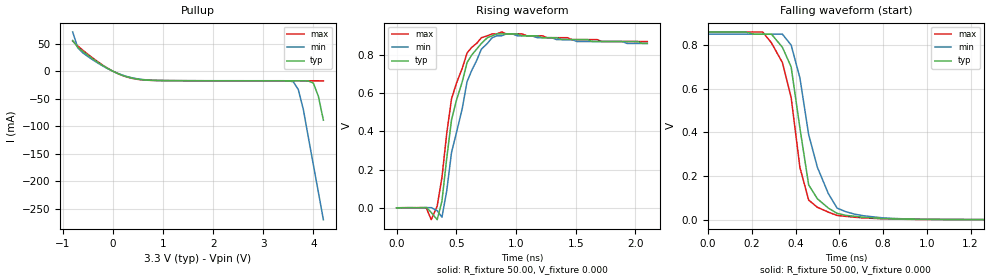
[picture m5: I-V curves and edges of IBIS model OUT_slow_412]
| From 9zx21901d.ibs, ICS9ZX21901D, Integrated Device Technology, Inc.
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|   Model OUT_slow_412
[Model]   OUT_slow_412
Model_type   Open_source
Polarity   Non-Inverting
Enable   Active-High
Vmeas =  0.350V
Cref =   2.00pF
Rref =  70.000
Vref =   0.350V
C_comp   3.40pF   2.85pF   3.95pF
[Temperature Range]   27.00   70.00   0.000
[Voltage Range]   3.30V   3.00V   3.60V
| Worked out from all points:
|   slope of the pullup table from 0 to 0.495 V, typ, clamps not added: 34.1 ohm
|   rising waveform, R_fixture 50.00, V_fixture 0.000: 20-80 % time 157ps typ, 172ps min, 146ps max; typ from 0.001 V to 0.86 V
|   falling waveform, R_fixture 50.00, V_fixture 0.000: 20-80 % time 76.4ps typ, 117ps min, 90ps max; typ from 0.86 V to 0.001 V
[Pullup]
| voltage   I(typ)   I(min)   I(max)
|  -3.30   2.07A   2.09A   2.05A
  |-3.10   1.90A   1.92A   1.88A
  |-2.90   1.73A   1.75A   1.71A
  |-2.70   1.56A   1.58A   1.54A
  |-2.50   1.39A   1.42A   1.37A
  |-2.30   1.22A   1.25A   1.20A
  |-2.10   1.05A   1.08A   1.03A
  |-1.90   0.89A   0.92A   0.87A
  |-1.70   0.72A   0.75A   0.70A
  |-1.50   0.56A   0.59A   0.53A
  |-1.00   0.16A   0.20A   0.14A
  |-0.90   96.58mA   0.13A   80.63mA
-800mV    56.17mA    71.66mA    55.16mA
-700mV    43.89mA    43.09mA    46.28mA
-600mV    36.41mA    33.82mA    38.59mA
0V        280uA      260uA      290uA
400mV     -12.7mA    -12.09mA   -13.11mA
900mV     -16.67mA   -16.56mA   -16.7mA
3.6V      -17.16mA   -18.93mA   -17.22mA
3.7V      -17.16mA   -33.24mA   -17.22mA
3.8V      -17.2mA    -69.35mA   -17.22mA
4V        -21.31mA   -170mA     -17.23mA
4.1V      -45.35mA   -220mA     -17.24mA
4.2V      -88.86mA   -270mA     -17.42mA
  | 4.30   -0.14A   -0.32A   -18.91mA
   |4.50   -0.25A   -0.43A   -72.19mA
   |4.70   -0.36A   -0.54A   -0.18A
   |4.90   -0.47A   -0.66A   -0.29A
   |5.10   -0.58A   -0.77A   -0.40A
   |5.30   -0.70A   -0.88A   -0.52A
   |5.50   -0.81A   -0.99A   -0.63A
   |5.70   -0.93A   -1.10A   -0.75A
   |5.90   -1.04A   -1.22A   -0.86A
   |6.10   -1.16A   -1.33A   -0.98A
   |6.60   -1.45A   -1.61A   -1.27A
[Ramp]
| variable   typ   min   max
dV/dt_r   0.52/0.16n   0.52/0.17n   0.52/0.16n
dV/dt_f   0.51/98.05p   0.51/0.11n   0.52/89.85p
R_load = 50.00
[Rising Waveform]
R_fixture = 50.00
V_fixture = 0.000
V_fixture_min = 0.000
V_fixture_max = 0.000
| time   V(typ)   V(min)   V(max)
0s        760uV      660uV      830uV
250ps     2.52mV     1.61mV     -1.52mV
290ps     -23.72mV   1.58mV     -61.26mV
340ps     -61.5mV    -14.51mV   9.86mV
380ps     35.89mV    -48.5mV    160mV
460ps     460mV      290mV      570mV
590ps     760mV      660mV      810mV
710ps     860mV      830mV      890mV
920ps     910mV      910mV      910mV
2.1ns     860mV      860mV      870mV
[Falling Waveform]
R_fixture = 50.00
V_fixture = 0.000
V_fixture_min = 0.000
V_fixture_max = 0.000
| time   V(typ)   V(min)   V(max)
0s        860mV      850mV      860mV
250ps     850mV      850mV      860mV
340ps     790mV      850mV      720mV
380ps     700mV      800mV      560mV
420ps     420mV      650mV      240mV
460ps     160mV      390mV      90.13mV
550ps     53.76mV    120mV      35.22mV
590ps     29.72mV    53.64mV    20.11mV
800ps     6.1mV      8.87mV     4.49mV
2.1ns     760uV      670uV      830uV
